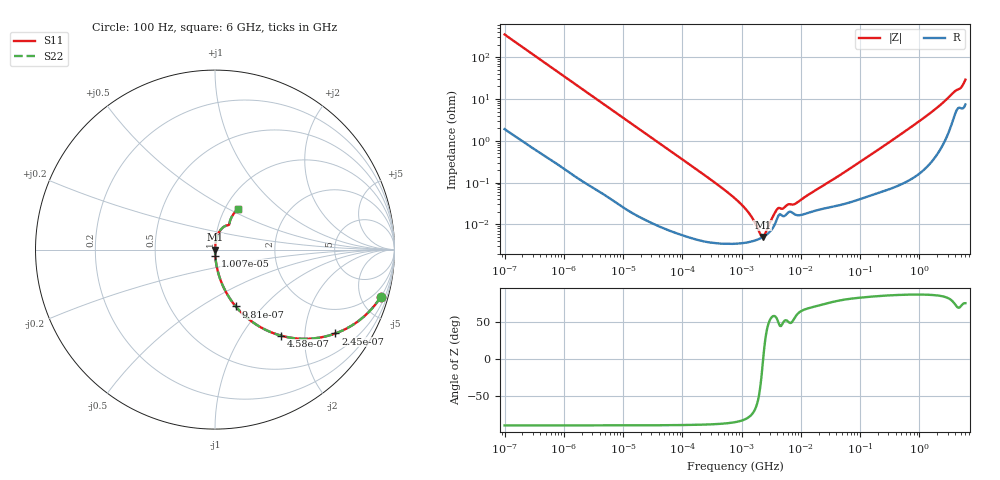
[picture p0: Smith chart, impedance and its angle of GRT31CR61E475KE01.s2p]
!Murata Part Number: GRT31CR61E475KE01
!These Parameters are Measured in Series Mode Connection
!Data Generated on Jun 19, 2026
!  o--ll--o
!Port1  Port2
!  o------o
!Operation Temp=25[degC], DC Bias Voltage=0[V]
!Freq. Start=100[Hz] Stop=6[GHz] 401[Steps]
# Hz S RI R 50
!Freq.(Hz) S11(Real) S11(Imag) S21(Real) S21(Imag) S12(Real) S12(Imag) S22(Real) S22(Imag)
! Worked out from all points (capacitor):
!   401 points, 100 Hz to 6 GHz, reference 50 ohm
!   read as one part in series: C = 4.55 uF near 109 Hz
!   lowest |Z| = 4.96 mohm at 2.269 MHz (marker M1)
!   series resonance near 2.315 MHz, so ESL is about 1 nH
!   S11 on the Smith chart (normalised r, x): 100 Hz: 1.04, -6.98; 245 Hz: 1.02, -2.86; 458 Hz: 1.01, -1.53; 981 Hz: 1.00, -0.72; 10.07 kHz: 1.00, -0.07; 6 GHz: 1.15, +0.56
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100  0.9229 -0.2641  0.0771 0.2641  0.0771 0.2641  0.9229 -0.2641
150  0.8436 -0.3604  0.1564 0.3604  0.1564 0.3604  0.8436 -0.3604
245  0.6705 -0.4672  0.3295 0.4672  0.3295 0.4672  0.6705 -0.4672
458  0.3701 -0.4799  0.6299 0.4799  0.6299 0.4799  0.3701 -0.4799
981  0.1154 -0.3165  0.8846 0.3165  0.8846 0.3165  0.1154 -0.3165
2008  0.0309 -0.17  0.9691 0.17  0.9691 0.17  0.0309 -0.17
10066  0.0015 -0.0352  0.9985 0.0352  0.9985 0.0352  0.0015 -0.0352
40335  0.000168 -0.00885  0.9998 0.00885  0.9998 0.00885  0.000168 -0.00885
316350  3.74e-05 -0.00112  1 0.00112  1 0.00112  3.74e-05 -0.00112
774597  3.44e-05 -0.000414  1 0.000414  1 0.000414  3.44e-05 -0.000414
1212075  3.67e-05 -0.000217  1 0.000217  1 0.000217  3.67e-05 -0.000217
1734173  4.16e-05 -9.24e-05  1 9.24e-05  1 9.24e-05  4.16e-05 -9.24e-05
2268635  4.92e-05 -6.4e-06  1 6.4e-06  1 6.4e-06  4.92e-05 -6.4e-06
2837864  6.16e-05 6.7e-05  0.9999 -6.7e-05  0.9999 -6.7e-05  6.16e-05 6.7e-05
4060267  0.000146 0.000187  0.9999 -0.000187  0.9999 -0.000187  0.000146 0.000187
7947587  0.000172 0.000255  0.9998 -0.000255  0.9998 -0.000255  0.000172 0.000255
1.555665e7  0.000202 0.000546  0.9998 -0.000546  0.9998 -0.000546  0.000202 0.000546
3.124326e8  0.000776 0.00922  0.9992 -0.00922  0.9992 -0.00922  0.000776 0.00922
2.048624e9  0.00888 0.0626  0.9911 -0.0626  0.9911 -0.0626  0.00888 0.0626
3.8344e9  0.0522 0.129  0.9478 -0.129  0.9478 -0.129  0.0522 0.129
5.016141e9  0.0816 0.1514  0.9184 -0.1514  0.9184 -0.1514  0.0816 0.1514
6e9  0.1278 0.2269  0.8722 -0.2269  0.8722 -0.2269  0.1278 0.2269
